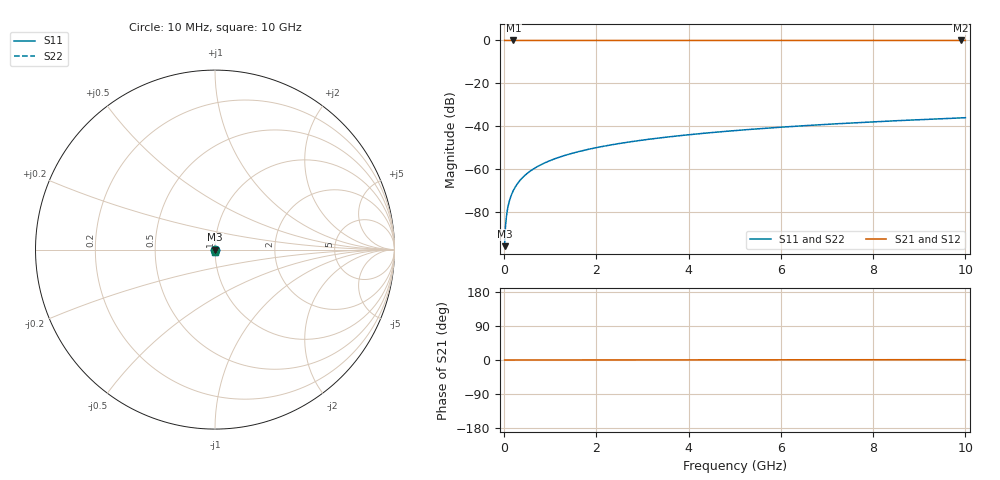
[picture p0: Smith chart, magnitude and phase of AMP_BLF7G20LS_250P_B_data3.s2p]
! AWR Design Environment (6079) Fri Apr 26 14:20:18 2013
! Simulator: Linear circuit simulator
! Ports: 2, Freqs: 1001
# GHz S MA R 50
!Freq  MagS11  AngS11  MagS21  AngS21  MagS12  AngS12  MagS22  AngS22
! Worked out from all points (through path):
!   1000 points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, 10 MHz to 10 GHz, reference 50 ohm
!   highest |S21| = 0.00 dB at 200 MHz (marker M1); lowest = 0.0 dB at 9.9 GHz (marker M2)
!   lowest |S11| = -96.1 dB at 10 MHz (marker M3), VSWR 1.00, Z = 50 - j0.00157 ohm
!   |S11| at or under -10 dB: start of sweep to end of sweep
!   |S22| runs from -96.1 to -36.1 dB; largest |S21 - S12| = 0
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0.01  1.571e-05 -90.0  1 0.0  1 0.0  1.571e-05 -90.0
0.04  6.283e-05 -90.0  1 0.0  1 0.0  6.283e-05 -90.0
0.07  0.00011 -90.0  1 0.0  1 0.0  0.00011 -90.0
0.1  0.0001571 -90.0  1 0.0  1 0.0  0.0001571 -90.0
0.15  0.0002356 -90.0  1 0.0  1 0.0  0.0002356 -90.0
0.2  0.0003142 -90.0  1 0.0  1 0.0  0.0003142 -90.0
0.28  0.0004398 -90.0  1 0.0  1 0.0  0.0004398 -90.0
0.39  0.0006126 -90.0  1 0.0  1 0.0  0.0006126 -90.0
0.53  0.0008325 -90.0  1 0.0  1 0.0  0.0008325 -90.0
0.69  0.001084 -89.9  1 0.1  1 0.1  0.001084 -89.9
0.88  0.001382 -89.9  1 0.1  1 0.1  0.001382 -89.9
1.11  0.001744 -89.9  1 0.1  1 0.1  0.001744 -89.9
1.38  0.002168 -89.9  1 0.1  1 0.1  0.002168 -89.9
1.68  0.002639 -89.8  1 0.2  1 0.2  0.002639 -89.8
2.41  0.003786 -89.8  1 0.2  1 0.2  0.003786 -89.8
3.34  0.005246 -89.7  1 0.3  1 0.3  0.005246 -89.7
4.12  0.006471 -89.6  1 0.4  1 0.4  0.006471 -89.6
5.01  0.007869 -89.5  1 0.5  1 0.5  0.007869 -89.5
6.67  0.01048 -89.4  1 0.6  1 0.6  0.01048 -89.4
8.34  0.0131 -89.2  0.9999 0.8  0.9999 0.8  0.0131 -89.2
9.9  0.01555 -89.1  0.9999 0.9  0.9999 0.9  0.01555 -89.1
10  0.01571 -89.1  0.9999 0.9  0.9999 0.9  0.01571 -89.1
